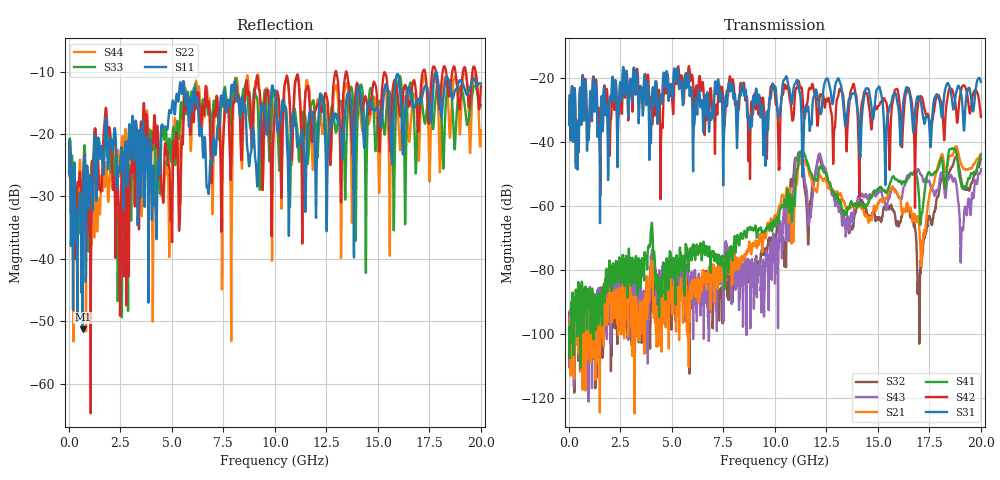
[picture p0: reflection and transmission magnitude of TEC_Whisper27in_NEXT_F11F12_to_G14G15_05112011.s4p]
! Tyco Electronics
! F11F12-G14G15_NEXT
!! PART DESCRIPTION: Whisper 27in Megtron 6 VLP-HVLP-VLP Channel Model, bulkhead 2.4mm test pts
!! MODEL DESCRIPTION: System 4-port S-parameter
!! MODEL STATUS: Measured
!! MODEL GEOMETRY: Channel Model
!! MODEL FREQUENCY RANGE: DC to 20.000 GHz in 10.000 MHz frequency steps
!! MODEL EDGE RATE LIMITATION: 25.00 ps (Using conservative 0.5/Fmax rule of thumb)
!! TIME-DOMAIN TRANSFORM CAUTIONS:
!! 1.) Do not simulate transient edge rates faster than the number listed above.  Edge rates faster than this number
!!  contain significant spectral content at frequencies above the model's highest frequency.
!! 2.) Even when simulating edge rates that are slower than the number listed above, be aware that the best time
!!  resolution possible with a direct iFFT is (1 / 2Fmax).  As a result, time resolution is typically not adequate
!!  for most time-domain simulations unless tricks such as windowing are used to minimize leakage and aliasing.
!! 3.) Because the model has a uniform frequency step, a direct iFFT will result in an impulse that that has a time
!!  length given by either (1 / Fstep) or (1 / 2Fstep), depending on the transform being used.  Care has been taken
!!  in selecting the frequency step to ensure a settled impulse response for the model.  Therefore, convolution with
!!  the model's impulse response should present no issues.  However, if directly concatenating s-parameter models
!!  in the frequency domain a user must either interpolate necessary interim frequencies or complete impulse response
!!  zero-padding.  Impulse response zero-padding is more difficult, but more accurate.
!! PORT DEFINITIONS:
!! Port  1  ----->  Side A  F11  G14  Side A  <-----  Port  2
!! Port  3  ----->  Side A  F12  G15  Side A  <-----  Port  4
! Point-to-Point link (differential)  !
! Connectors:  !
!  1: STRADA Whisper  !
! Materials:  !
!  Backplane: Megtron-6 HVLP  !
!  Daughtercard: Megtron-6 VLP  !
! Stack-up:  !
!  Backplane: 20 layers, 200mil thick  !
!  Daughtercard: 14 layers, 110mil thick  !
! Trace Length:  !
!  Backplane: 17in  !
!  Daightercards: 5in  !
! Trace Width:  !
!  Backplane: 8-13-8 mils  !
!  Daughtercards: 6-9-6 mils  !
! Geometry:  !
!  Backplane: Stripline  !
!  Daughtercards: Stripline  !
! Freq. Range: 0 GHz - 20 GHz  !
! Note1: non-mixed-mode s-parameters  !
! Note2: channel includes 2.4mm test points  !
! Created Wed May 11 15:01:32 2011
! 4 Port Network Data from SP1.SP block
! freq  magS11  angS11  magS12  angS12  magS13  angS13  magS14  angS14
!  magS21  angS21  magS22  angS22  magS23  angS23  magS24  angS24
!  magS31  angS31  magS32  angS32  magS33  angS33  magS34  angS34
!  magS41  angS41  magS42  angS42  magS43  angS43  magS44  angS44
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# hz S ma R 50
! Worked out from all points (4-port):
!   2000 points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, 10 MHz to 20 GHz, reference 50 ohm
!   strongest paths, dB at 10 MHz, 5.01 GHz, 10.01 GHz, 15.01 GHz, 20 GHz:
!     S31: -34.6, -25.5, -22.6, -23.0, -21.2
!     S42: -34.5, -26.7, -25.9, -28.7, -32.1
!     S41: -106.8, -81.4, -66.3, -54.7, -44.0
!     S21: -100.6, -91.5, -62.8, -59.3, -43.7
!     S43: -94.4, -89.9, -82.9, -55.7, -48.5
!     S32: -108.0, -90.7, -72.5, -64.2, -45.2
!   lowest |S11| = -51.3 dB at 670 MHz (marker M1), VSWR 1.01, Z = 49.8 + j0.117 ohm
!   |S11| at or under -10 dB: start of sweep to 17.81 GHz; 17.83 GHz to end of sweep
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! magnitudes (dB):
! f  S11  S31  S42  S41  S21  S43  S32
! 10 MHz  -26.4  -34.6  -34.5  -106.8  -100.6  -94.4  -108.0
! 670 MHz  -51.3  -19.3  -19.0  -86.1  -117.6  -88.7  -97.8
! 9.43 GHz  -16.1  -42.1  -26.4  -67.9  -70.8  -78.5  -75.4
! 11.09 GHz  -22.1  -20.6  -22.6  -48.5  -51.3  -45.6  -44.9
! 17 GHz  -14.5  -26.0  -26.2  -57.3  -66.5  -49.0  -89.0
! 19.07 GHz  -11.6  -26.1  -23.0  -53.8  -47.3  -67.8  -52.6
! 20 GHz  -11.9  -21.2  -32.1  -44.0  -43.7  -48.5  -45.2
